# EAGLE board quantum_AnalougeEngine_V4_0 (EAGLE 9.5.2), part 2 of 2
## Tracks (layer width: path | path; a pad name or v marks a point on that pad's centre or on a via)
0,5V_DAC  (via drill 0.5)
  Top(V+) 0.508: R61.1 R60.2 52.5,40 v51.8,39.3 | IC7.3 37.84,8.06 39.1,6.79 IC7.5 41.15,6.05 41.3,5.9 v44.4,5.9
  Bottom 0.508: v51.8,39.3 51.8,13.3 v44.4,5.9
1V_DAC
  Top(V+) 0.254: IC2.7 62.35,22.5
  Top(V+) 0.305: 62.35,22.5 C23.1 | IC3.7 62.35,11.7 C24.1
  Top(V+) 0.508: C34.1 63.85,11.65 C24.1 62.3,11.75 62.3,18.7 62.5,18.9 67.3,18.9 67.3,24 67,24.3 C33.1 63.85,22.55 C23.1 | C32.1 62.35,28.15 | 62.35,28.15 62.35,22.5 | 62.35,28.15 R68.1 64.65,33.6 C20.1 R69.2 64.75,36.3 R61.2
2V_DAC_REF
  Top(V+) 0.508: R67.1 60.65,34.8 | 60.65,34.8 R68.2 | 60.65,34.8 60.62,34.77 Z1.1
+3V3_STM32  (via drill 0.5)
  Top(V+) 0.406: R1.2 100.4,56.85 100.4,85 103.8,88.4 111.9,88.4 132.3,68 163.9,68 v164,68.1
  midBottom(V-) 0.406: v164,68.1 169.7,68.1 170.2,67.6 170.2,25.6 169.5,24.9 167.12,24.9 U1.CN11_16
+5V_STM32  (via drill 0.5)
  Top(V+) 0.2: C43.1 59.3,14.65 58.6,15.35 58.6,17.6 59,18 v59.5,18
  Top(V+) 0.254: IC3.1 55.3,15 55.3,15.4 C44.1
  Top(V+) 0.305: IC2.1 55.3,25.75 55.3,26.4 C31.1
  Top(V+) 0.406: C19.1 59.4,25.75 v58,25.75 55.3,25.75 | C43.1 59.15,15 55.3,15
  pour midTop(AGND): 53.1,31.9 53.1,-1.6 173.7,-1.6 173.7,108.6 100.9,108.6 100.9,48.2 91.7,48.2 91.7,6.7 60.8,6.7 60.8,31.9
+12V  (via drill 0.5)
  Top(V+) 0.406: U$1.3 C102.1 136.95,3.85 140.25,7.15 158.35,7.15 161.4,4.1 169.9,4.1 170.4,4.6 170.4,34.3 | 165.29,35 161.5,35 160.73,34.23 U1.CN8_15 | 170.4,34.3 169.7,35 165.29,35 | 170.4,34.3 170.4,96.7 170.2,96.9 163.3,96.9 155.34,88.94 U12.9
  Top(V+) 0.508: L2.2 10.8,72.42 K2.1 12.18,73.38 v12.2,73.4 | L4.2 36.1,72.42 K3.1 35.17,73.4 v38,73.4 | L1.2 60.4,72.52 K1.1 61.78,73.38 v61.8,73.4 | L3.2 85.8,72.42 K4.1 87.38,73.38 v87.4,73.4 | K5.1 85.8,48.22 L5.2 v87.6,46.7 | L6.2 10.8,54.77 K6.1 12.13,55.73 v12.2,55.8 | L7.2 23.4,54.77 K7.1 24.67,55.73 v24.7,55.7 | L8.2 36.2,54.77 K8.1 35.27,55.7 v37.7,55.7 | v99.6,96.5 146.6,96.5 U12.9 | 165.29,35
  midBottom(V-) 0.508: v37.7,55.7 v24.7,55.7 24.6,55.8 v12.2,55.8 v12.2,73.4 v38,73.4 v61.8,73.4 v87.4,73.4 99.6,73.4 100.4,74.2 | v99.6,96.5 100.4,95.7 100.4,74.2 | 100.4,74.2 100.4,54.2 98.3,52.1 76,52.1 75.4,51.5 75.4,45.4 75.9,44.9 87.7,44.9 88.2,45.4 88.2,46.1 v87.6,46.7
.  (via drill 0.5)
  Top(V+) 0.508: IC7.7 43.09,9.34 R72.2 v43.1,11.1 | v42.95,40.25 42,40.25 R59.2
  midBottom(V-) 0.508: v43.1,11.1 43.1,21.27 43.05,21.33 43.05,40.25 v42.95,40.25
...  (via drill 0.5)
  Top(V+) 0.508: IC7.1 33.76,10.61 R71.2 33.8,10.65 v33.8,11.9 | v43.1,48.2 R73.2
  midBottom(V-) 0.508: v33.8,11.9 35.8,13.9 41.6,13.9 42,14.3 42,47.1 v43.1,48.2
ADC1-IN0  (via drill 0.5)
  Top(V+) 0.254: R4.2 R3.1 95.75,61.55 v96.8,62.6
  Bottom 0.254: v96.8,62.6 96.87,62.6 97.18,62.92
  Bottom 0.406: 97.18,62.92 116.02,62.92 116.1,63 169.1,63 169.9,62.2 169.9,40.5 169.56,40.16 166.88,40.16 165.81,39.08 U1.CN11_28
ADC1-IN3  (via drill 0.5)
  Top(V+) 0.254: R2.2 R1.1 v94.2,53.9
  Bottom 0.254: v94.2,53.9 94.2,58.8 97.6,62.2
  Bottom 0.406: 97.6,62.2 101.6,62.2 103.4,60.4 118.5,60.4 118.5,54.3 117,52.8 108.66,52.8 U1.CN12_37
AGND  (via drill 0.5)
  Top(V+) 0.254: R4.1 v98.7,60.2 | C22.2 v98.7,64.5
  Top(V+) 0.305: R6.1 R15.1 R16.1 R23.1 R24.1 | R24.1 R25.1 R26.1 R27.1 | R24.1 78.05,25.9 77.06,26.89 U$4.G6 | R39.1 v43.7,34.3 | R42.1 v43.7,30.1 | R45.1 v43.7,25.9 | R65.1 43.7,21.7 v43.7,21.6
  Top(V+) 0.406: OUT_LEFT.3 42.06,86.36 v42.1,86.4 | C12.2 38.6,80.55 | 40.65,75.25 v40.6,75.2 | TP04.P$1 CONN3.1 21.89,7.7 10.1,7.7 +15VOK.1 10,8.8 9.9,8.9 7.7,8.9 5.6,6.8 3.11,6.8 2.31,7.6 2.31,12.01 3,12.7 5,12.7 5.35,12.35 R14.2
  Top(V+) 0.508: OUT_RIGHT.3 17.57,82.77 v17.5,82.7 | C14.2 v14.2,81.5 | C13.2 16.15,75.35 v16.1,75.3 | 38.6,80.55 v38.6,82 | C11.2 40.65,75.25 | IN_LEFT.1 v88.9,82.1 | C1.2 98.5,83 v99.3,83.8 | C3.2 73.7,83.23 v74.14,83.66 | IN_RIGHT.1 v64,81.81 v64,81.8 | C4.2 v63.8,75.1 | C2.2 v88.6,75 | C6.2 88.12,67.62 | 88.12,67.62 88.8,66.95 C21.2 | 88.12,67.62 88.23,67.73 v88.7,67.73 U4.2 | C26.2 v75.15,65.85 75.25,65.75 C5.2 | U6.1 64,69 v63.9,68.9 C25.2 | v47.6,59.8 C60.2 | C62.2 48.7,63.6 | 48.7,63.6 v47.6,63.6 | C63.2 v47.6,68.1 | C61.2 48.8,55.2 | 48.8,55.2 v47.6,55.2 | 48.8,55.2 50.23,56.63 VCA2(RIGHT).6 VCA2(RIGHT).3 | 48.7,63.6 50.03,64.94 VCA1(LEFT).6 VCA1(LEFT).3 | IC8.3 54.53,46.37 v55.35,45.55 55.8,45.09 IC8.5 | C54.2 v47.8,45.5 | C53.2 v63.4,48.7 | STAGE(RIGHT).3 STAGE(RIGHT).6 25.59,38.73 25.25,38.4 C46.2 v23.5,37.5 | STAGE(LEFT).3 STAGE(LEFT).6 25.68,46.84 25.15,46.3 C47.2 v23.4,45.5 | C48.2 v23.5,50 | C45.2 v23.5,41.9 | IC5.3 30.54,29.27 v31.8,28 IC5.5 | C36.2 v23.8,28 | C30.2 3.25,34.7 v4.3,34.7 | C28.2 13.35,34.5 v14.1,34.5 | C8.2 v12.8,31.5 | U7.2 7.96,37.47 v7.9,37.4 | v17.1,42 C29.2 | C27.2 v7.5,42 | C7.2 v24.4,24.7 | U8.1 v19.6,35 | R35.1 62.45,8.6 62.45,9.9 C24.2 v63.6,9.95 65.55,9.95 C34.2 | C23.2 v63.7,20.85 65.55,20.85 C33.2 | C32.2 66.45,29.15 v66.45,32 C20.2 R69.1 66.4,35.75 66.4,35.9 67.4,36.9 67.4,39.35 66.75,40 R60.1 | TP16.P$1 56.02,34 56.8,33.23 Z1.2 | C40.2 v37,16.3 | C39.2 v37,22.2 | C57.2 v27,17.8 | C58.2 27,24.6 v26.9,24.7 | C35.2 38.9,31.8 v39,31.9 | R46.1 v43.1,50.3 | R58.1 v42.95,42.5 | C49.2 v38.2,12.2 | C50.2 v38.6,5.2 | R47.1 R76.1 R65.1
  pour midTop(AGND): 91.1,7.5 61.5,7.5 61.5,32.7 52.5,32.7 52.5,-1.7 -1,-1.7 -1,108.4 100,108.4 100,49 91.1,49
BOTTOM
  pour Bottom: -1.7,-2.6 -1.7,109.2 174.4,109.2 174.4,-2.6
BUSY
  Top(V+) 0.406: U$4.BUSY 97.61,18 99.9,18 102.9,21 102.9,23.9 103.9,24.9 109.3,24.9 109.8,25.4 109.8,27.3 111.2,28.7 116.1,28.7 118.05,30.65 126.69,30.65 153.94,57.9 163.06,57.9 164.31,59.15 U1.CN11_44
CHASIS  (via drill 0.5)
  Top(V+) 0.406: C15.1 67.8,85.15 v67.8,88 | C18.1 92.75,87.85 v92.6,88
  Top(V+) 1.016: R77.1 50.3,7.9 48.9,6.5 TP03.P$1
  Bottom 1.016: 82.69,88 v92.6,88 | 82.69,88 73.89,96.8 40.2,96.8 OUT2(L/M).G OUT1(R/S).G 5.4,94.8 1.5,90.9 1.5,55.6 6.11,50.99 6.11,45.81 1.9,41.6 1.9,12.6 11.6,2.9 46.8,2.9 TP03.P$1 | 82.69,88 v67.8,88
CS  (via drill 0.5)
  Top(V+) 0.406: U$4.CS 100.53,16.73 103.6,19.8 109.3,19.8 110.6,21.1 110.6,25.3 111.4,26.1 115.7,26.1 119.34,29.74 127.14,29.74 152.7,55.3 162.2,55.3 163.1,56.2 v163.1,57
  Bottom 0.406: v163.1,57 163.1,59 164.46,60.36 167.08,60.36 168.35,61.64 U1.CN11_45
CS_DAC1  (via drill 0.5)
  Top(V+) 0.254: IC2.9 57.9,23.5 v57.3,24.1
  midBottom(V-) 0.305: v57.3,24.1 58,23.4 58,21.3 56.7,20 56.7,6.39 58.39,4.7
  midBottom(V-) 0.406: 58.39,4.7 93.01,4.7 93.88,5.57 93.88,11.98 94.9,13 99.5,13 102.7,16.2 102.7,31.8 103.4,32.5 109.9,32.5 110.8,33.4 110.8,41.4 109.6,42.6 103.4,42.6 102.9,42.1 102.9,40.5 103.3,40.1 106.4,40.1 107.39,39.11 U1.CN12_27
CS_DAC2  (via drill 0.5)
  Top(V+) 0.254: IC3.9 57.8,12.7 v57.4,13.1
  midBottom(V-) 0.305: v57.4,13.1 57.4,7 59,5.4
  midBottom(V-) 0.406: U1.CN12_29 109.13,41.37 109.6,40.9 109.6,35.9 108.8,35.1 103.8,35.1 101.6,32.9 101.6,17.6 99.5,15.5 93.9,15.5 92.9,14.5 92.9,5.9 92.4,5.4 59,5.4
CV_A_B
  Bottom 0.406: U1.CN11_3 168.35,8.55 167.3,9.6 163.7,9.6 159.91,13.39 111.01,13.39 109.7,14.7 101.54,14.7 99.81,12.96 97.65,12.96 U$4.CVB U$4.CVA
DAC2_OUT1(OFFSET_VCA1)  (via drill 0.5)
  Top(V+) 0.508: R76.2 R74.2 48.2,19.75 v48.2,21 | C39.1 v40.4,22.3 | v26.9,20.1 26.43,20.57 IC9.3
  Bottom 0.508: v48.2,21 46.95,22.25 40.45,22.25 v40.4,22.3 38.2,20.1 v26.9,20.1
DAC2_OUT2(OFFSET_VCA2)  (via drill 0.5)
  Top(V+) 0.508: R47.2 R75.2 48.1,17.45 v48.1,15.8 | v40.4,16.5 C40.1 38.8,19.9 35.6,19.9 34.99,19.3 IC9.5
  Bottom 0.508: v40.4,16.5 40.5,16.6 47.3,16.6 v48.1,15.8
DAC2_OUT3
  Top(V+) 0.254: IC3.4 45.8,11.7 43.9,13.6 34.65,13.6 R62.1
DAC2_OUT4
  Top(V+) 0.254: IC3.5 45.75,11.2 45.3,10.75 R70.1
DAC_OUT1  (via drill 0.5)
  Top(V+) 0.508: R57.1 18.25,23.05 v18.2,23
  midBottom(V-) 0.406: v18.2,23 18.2,20.2 27.5,10.9 27.5,3.8 29.6,1.7 116.1,1.7 157.1,42.7 164.6,42.7 U1.CN11_32
DAC_OUT2  (via drill 0.5)
  Top(V+) 0.508: R55.1 34.85,22.25 v34.9,22.3
  midTop(AGND) 0.406: v110.3,5.8 110.3,17.6 109.39,18.51 U1.CN12_11
  midBottom(V-) 0.406: v34.9,22.3 34.9,16.7 29.1,10.9 29.1,3.9 30.1,2.9 107.5,2.9 110.3,5.7 v110.3,5.8
DB0
  midBottom(V-) 0.406: U$4.DB0 97.57,20.5 94.8,20.5 94.2,21.1 94.2,42.94 97.51,46.25 102.05,46.25 102.7,46.9 102.7,83.5 103.75,84.55 U1.CN12_64 105.41,84.55 106.69,83.27 109.63,83.27 115.01,77.89 U1.CN10_33
DB1
  midBottom(V-) 0.406: U$4.DB1 97.6,23.07 97.6,43.1 99.7,45.2 126.6,45.2 164.7,83.3 167.06,83.3 U1.CN11_61
DB2
  midTop(AGND) 0.406: U$4.DB2 101.25,24.35 102.2,25.3 102.2,26.9 102.69,27.39 108.89,27.39 109.67,28.16 109.67,31.77 110.2,32.3 117,32.3 117,63.7 116.47,64.23 U1.CN10_25 145.53,64.23 155.69,54.07 U1.CN9_14
DB3
  Top(V+) 0.406: U$4.DB3 97.59,25.6 99.9,25.6 100.7,26.4 100.7,28.7 101.9,29.9 108.6,29.9 109.1,30.4 109.1,31.6 109.8,32.3 124.3,32.3 156.3,64.3 158.12,64.3 U1.CN9_22 159.46,65.5 167.08,65.5 U1.CN11_47
DB4
  Bottom 0.406: U$4.DB4 102.01,26.89 104,24.9 109.1,24.9 110.6,26.4 110.6,28.1 111.24,28.74 116.14,28.74 117.94,30.54 126.54,30.54 152.6,56.6 U1.CN9_16
DB5
  Bottom 0.406: U$4.DB5 96.34,26.9 97.56,28.12 102.5,28.12 103.18,27.44 109.04,27.44 109.8,28.2 109.8,30.5 110.75,31.45 126.09,31.45 153.79,59.15 U1.CN9_18
DB6
  midBottom(V-) 0.406: U1.CN9_20 159.5,63 162.8,63 162.8,79.8 165.01,82.01 U1.CN11_62
  Bottom 0.406: U$4.DB6 98.93,29.43 99.4,29.9 108.5,29.9 109,30.4 109,31.8 109.6,32.4 125.8,32.4 155.1,61.7 U1.CN9_20
DB7
  Bottom 0.406: U$4.DB7 97.51,30.6 100.2,30.6 101.3,31.7 101.3,59.4 104.6,59.4 U1.CN12_44 106.1,57.9 111.18,57.9 U1.CN10_20
DB8
  midTop(AGND) 0.406: U$4.DB8 102.9,35.99 102.9,55.3 111.24,55.3 U1.CN10_18
DB9  (via drill 0.5)
  Top(V+) 0.406: U$4.DB9 97.57,33.2 100.4,33.2 101,33.8 101,36.4 102.2,37.6 111.16,37.6 U1.CN10_4 112.47,36.47 113.6,37.6 117.6,37.6 118.7,38.7 v118.7,47.1
  midBottom(V-) 0.406: U1.CN12_52 105.29,69.31 106.6,68 115.8,68 118.6,65.2 118.6,47.2 v118.7,47.1
DB10
  midTop(AGND) 0.406: U$4.DB10 102,37.63 102,65.51 106.11,65.51 U1.CN12_47 109.83,64.23 112.37,61.69 U1.CN10_24
DB11
  Top(V+) 0.406: U1.CN10_6 112.47,38.84 111.16,40.16 101.56,40.16 101.1,39.7 101.1,37.4 99.44,35.74 97.57,35.74 U$4.DB11
DB12
  midTop(AGND) 0.406: U$4.DB12 101.3,39.47 101.3,68.1 106.06,68.1 107.28,66.88 | 107.28,66.88 U1.CN12_49 | U1.CN10_26 109.82,66.88 107.28,66.88
DB13
  Top(V+) 0.406: U$4.DB13 97.55,38.26 99.31,38.26 100.3,39.26 100.3,44.7 100.84,45.24 111.14,45.24 U1.CN10_10 112.47,44.06 113.64,45.24 116.94,45.24 117.8,46.1 117.8,74.3 115.7,76.4 109.4,76.4 U1.CN12_55
DB14
  Top(V+) 0.406: U$4.DB14 98.88,44.79 102.05,47.96 102.05,69.9 102.69,70.54 106.16,70.54 U1.CN12_51 107.45,69.37 109.87,69.37 U1.CN10_28
DB15
  Top(V+) 0.406: U$4.DB15 96.34,43.39 101.4,48.45 101.4,71.6 102.98,73.18 106.06,73.18 U1.CN12_53
DGND
  pour Top(V+): 53.1,31.9 53.1,-1.2 173.4,-1.2 173.4,108.6 100.9,108.6 100.9,48.2 91.7,48.2 91.7,6.6 61.1,6.6 61.1,31.9
  pour midBottom(V-): 53,31.9 53,-2.1 174.1,-2.1 174.1,108.6 100.9,108.6 100.9,48.2 91.7,48.2 91.7,6.6 60.8,6.6 60.8,31.9
DIN_DAC  (via drill 0.5)
  Top(V+) 0.254: IC3.8 58.4,12.2 56.1,9.9 v56.1,9.8
  Top(V+) 0.305: IC2.8 57.8,23 v57.2,22.4
  midBottom(V-) 0.305: v57.2,22.4 56.1,21.3 v56.1,9.8 56.1,5.7 57.8,4
  midBottom(V-) 0.406: 57.8,4 93.6,4 94.8,5.2 94.8,10.1 95,10.3 99.5,10.3 103.9,14.7 109.8,14.7 110.8,15.7 110.8,17.8 111.5,18.5 129.7,18.5 156.4,45.2 160.1,45.2 160.73,44.57 U1.CN9_5
E+_OUT_STAGE_LEFT
  Top(V+) 0.508: STAGE(LEFT).2 37.77,45.56 38.3,46.1 TP02.P$1 40.05,48.8 40.15,48.9 | R46.2 40.15,48.9 | 40.15,48.9 R73.1
E+_OUT_STAGE_RIGHT
  Top(V+) 0.508: STAGE(RIGHT).2 37.27,37.47 38.2,38.4 TP01.P$1 39.95,41 40.15,41.2 | R58.2 40.15,41.2 | 40.15,41.2 R59.1
EC+_VCA1(LFT)  (via drill 0.5)
  Top(V+) 0.508: VCA1(LEFT).2 60.06,63.66 60.85,64.45 TP37.P$1 60.85,68.55 60,69.4 v45,69.4 | R56.2 24.09,23.05 IC9.1 26.2,23.11 v27.4,21.9
  Bottom 0.508: v27.4,21.9 30.5,21.9 33.19,24.59 33.19,48.19 43.7,58.7 43.7,68.1 v45,69.4
EC+_VCA2(RIGHT)  (via drill 0.5)
  Top(V+) 0.508: VCA2(RIGHT).2 59.97,55.37 60.85,56.25 TP36.P$1 57.95,60.8 v45.5,60.8 | IC9.7 31.39,21.84 R54.2 33.15,23.6 v34.2,23.6
  Bottom 0.508: v34.2,23.6 34.2,47.7 44.7,58.2 44.7,60.4 45.1,60.8 v45.5,60.8
FRST
  Top(V+) 0.406: U$4.FRST 97.67,20.6 100.4,20.6 101.6,21.8 101.6,26 103,27.4 108.5,27.4 109.9,28.8 109.9,30.7 110.7,31.5 126,31.5 154.88,60.38 167.62,60.38 168.35,59.65 U1.CN11_43
L  (via drill 0.5)
  Top(V+) 0.508: IN_LEFT.6 IN_LEFT.5 96.2,72.9 95.3,72 90.92,72 88.77,69.85 82.92,69.85 82.4,69.33 v82.4,68.3 82.45,68.3 82.45,67.33 82.64,67.14 IC4.3 | v82.4,54.3 84.9,54.3 K5.Q1
  Bottom 0.508: v82.4,68.3 v82.4,54.3
L/M_IN(VCA1_IN)
  Top(V+) 0.508: C67.1 71.8,60.7 74.4,58.1 80.7,58.1 82,56.8 K5.P1 88,56.8 90.2,54.6 90.2,42.55 87.25,39.6 R5.1
L/M_OUT(OUT_STAGE_LEFT)  (via drill 0.5)
  Top(V+) 0.305: R19.1 88.3,25.9 90.3,23.9 90.3,13.7 88.1,11.5 71.5,11.5 68.3,14.7 68.3,40.4 67.4,41.3 47.4,41.3 40.1,34 28.7,34 26.8,32.1 R28.2
  Top(V+) 0.508: IC5.1 27.36,31.8 R28.2 C37.2 23.95,31.25 | IC1.3 18.86,29.54 19.3,29.1 21.8,29.1 23.95,31.25 | 23.95,31.25 22.4,32.8 v22.4,35.3 | v9.8,59.2 9.8,60.86 K6.Q1
  Bottom 0.508: v22.4,35.3 15.4,42.3 15.4,59.2 v9.8,59.2
L/M_OUT(VCA1_OUT)  (via drill 0.5)
  Top(V+) 0.508: 52.5,48.91 50.76,48.91 R48.2 C55.2 48.6,48.85 45.55,48.85 43.9,47.2 43.9,45.5 42.7,44.3 R36.1 | 52.5,48.91 IC8.1 | R17.1 86.55,32.8 88.5,34.75 v88.5,37.9 | v52.6,50.1 52.6,49.01 52.5,48.91
  Bottom 0.508: v88.5,37.9 88.5,41.2 86.6,43.1 54.1,43.1 52.6,44.6 v52.6,50.1
L/M_OUT+
  Top(V+) 0.508: K3.S1 36.66,83.64 37.4,82.9 37.4,75.6 39,74 44.6,74 OUT_LEFT.8 | OUT_LEFT.8 OUT_LEFT.7 | OUT_LEFT.8
L/M_OUT-
  Top(V+) 0.508: K3.S2 30.14,83.64 33.9,87.4 44,87.4 44,84.6 | OUT_LEFT.2 44,84.6 | 44,84.6 OUT_LEFT.1
M
  Top(V+) 0.508: U4.5 U4.6 96.3,63.52 92.12,59.34 K5.S1
M1  (via drill 0.5)
  Top(V+) 0.508: U7.6 U7.5 v4.6,42.4 | K6.S1 7.99,65.99 v7.6,65.6
  Bottom 0.508: v7.6,65.6 8.8,64.4 8.8,44.5 6.7,42.4 v4.6,42.4
N$1
  Top(V+) 0.406: C9.1 63.05,81.25 63.77,80.53 IN_RIGHT.2
  Top(V+) 0.508: C9.1 63.05,83.64 K1.S1
N$2
  Top(V+) 0.508: K1.S2 53.36,83.64 57.2,79.8 63,79.8 63.53,79.27 IN_RIGHT.3 68.3,79.27 68.3,81.3 69.9,82.9 72.03,82.9 73.45,84.33 73.45,84.6 C10.2
N$3
  Top(V+) 0.406: C9.2 66.35,83.5 69.2,83.5 69.55,83.85 C15.2 C10.1
N$4  (via drill 0.5)
  Top(V+) 0.305: U$4.V1 72.24,39.59 73.59,40.94 75.51,40.94 76.5,39.95 76.5,38.65 v76.35,38.5 | v83.1,38 83.1,38.95 | 83.1,38.95 R5.2 | 83.1,38.95 82.45,39.6 R6.2
  Bottom 0.305: v76.35,38.5 82.6,38.5 v83.1,38
N$5
  Top(V+) 0.508: K8.Q1 33.13,60.91 30.23,58 29.1,58 26,58 24.4,59.6 19.97,59.6 18.99,60.58 18.99,66 | 18.99,66 22.43,66 K7.S1 | 18.99,66 18.99,66.01 17.55,67.45 8.05,67.45 6.6,66 6.6,64.1 7.25,63.45 K6.P1
N$6  (via drill 0.5)
  Top(V+) 0.305: U$4.V2 71.34,37.05 70.96,37.43 70.96,40.25 72.36,41.65 75.9,41.65 77.2,40.34 77.2,34.95 v77.06,34.8 | v83.1,34.4 83.1,35.75 | 83.1,35.75 83.05,35.7 R15.2 | 83.1,35.75 R13.2
  Bottom 0.305: v77.06,34.8 82.7,34.8 v83.1,34.4
N$7
  Top(V+) 0.508: K4.S2 79.78,83.64 80.4,83.02 80.4,80.7 81.21,79.89 88.51,79.89 88.9,79.5 90.94,79.5 IN_LEFT.3 93.06,79.56 93.9,80.4 93.9,82.5 95,83.6 97.33,83.6 98.65,84.92 C17.2
N$8  (via drill 0.5)
  Top(V+) 0.508: K2.Q1 7.66,78.56 v6.7,77.6 | v59.25,76.45 59.25,78.26 K1.Q1
  Bottom 0.508: v6.7,77.6 14.9,77.6 58.2,77.6 59.3,76.5 v59.25,76.45
N$9
  Top(V+) 0.406: C17.1 C18.2 94.45,84.3 94.25,84.1 91.95,84.1 90.95,85.1 C16.2
N$10  (via drill 0.5)
  Top(V+) 0.305: U$4.V3 70.84,34.51 70.35,34.99 70.35,40.64 72.06,42.35 76.39,42.35 77.91,40.84 77.91,31.45 v77.76,31.3 | v83.1,30.9 83.1,32.05 | 83.1,32.05 83.1,32.15 R17.2 | 83.1,32.05 R16.2
  Bottom 0.305: v77.76,31.3 82.7,31.3 v83.1,30.9
N$11  (via drill 0.5)
  Top(V+) 0.508: K2.Q2 4.51,76.6 v9.8,76.6 | v52,76.6 52,78.3 K1.Q2
  Bottom 0.508: v9.8,76.6 v52,76.6
N$12  (via drill 0.5)
  Top(V+) 0.305: U$4.V4 70.98,31.97 69.65,33.3 69.65,40.93 71.77,43.06 76.99,43.06 78.61,41.43 78.61,28.21 v78.3,27.9 | v83.1,27.5 83.1,28.75 | 83.1,28.75 R18.2 | 83.1,28.75 82.45,29.4 R23.2
  Bottom 0.305: v78.3,27.9 82.7,27.9 v83.1,27.5
N$13
  Top(V+) 0.406: C16.1 88.05,85.1 87.95,85 87.95,81.35 88.5,80.8 90.97,80.8 IN_LEFT.2
  Top(V+) 0.508: C16.1 85.2,85.1 84.84,84.75 K4.S1
N$14
  Top(V+) 0.508: L1.1 53.25,71.3 R7.2
N$15  (via drill 0.5)
  Top(V+) 0.508: v32,81.1 K3.P1
  Bottom 0.508: OUT2(L/M).3 32,83.52 v32,81.1
N$16
  Top(V+) 0.508: R8.2 84.1,71.1 L3.1
N$17  (via drill 0.5)
  Top(V+) 0.508: K3.P2 v30.4,81.1
  Bottom 0.508: v30.4,81.1 30.4,85.73 OUT2(L/M).2
N$18  (via drill 0.5)
  Top(V+) 0.508: U4.3 92.64,66.47 93.4,65.7 93.4,64.5 92.1,63.2 84.75,63.2 84.05,63.9 IC4.1 IC4.2 81.83,65.86 81.05,66.65 81.05,68.8 80.45,69.4 v76.6,69.4 | U6.2 66.23,67.7 v67.9,67.7
  Bottom 0.508: v76.6,69.4 69.6,69.4 v67.9,67.7
N$19
  Top(V+) 0.508: K8.S1 32.84,65.99 32.24,65.39 32.24,61.39 29.96,59.11 26.25,59.11 24.45,60.91 K7.Q1 20.39,60.91 20,61.3 20,64.1 20.66,64.75 24.29,64.75 24.69,65.15 24.69,67 24.4,67.29 19.05,67.29 17.93,68.4 7.72,68.4 5.6,66.28 5.6,64.2 4.85,63.45 K6.P2
N$20  (via drill 0.5)
  Top(V+) 0.305: U$4.V5 70.94,29.43 69.65,28.14 69.65,15.87 71.77,13.74 76.59,13.74 78.3,15.46 v78.3,24.4 | v83.1,24 83.1,25.25 | 83.1,25.25 R19.2 | 83.1,25.25 82.45,25.9 R24.2
  Bottom 0.305: v83.1,24 82.7,24.4 v78.3,24.4
N$21
  Top(V+) 0.508: IN1(R/S).2 65.64,92.5 57.12,92.5 55.49,90.88 55.49,86.49 54.1,85.1 50.71,85.1 49.8,84.19 49.8,81.6 50.3,81.1 K1.P2
N$22
  Top(V+) 0.508: IN1(R/S).3 57.95,90.35 57.1,89.5 57.1,81.6 57.6,81.1 K1.P1
N$23  (via drill 0.5)
  Top(V+) 0.508: v5.6,81.1 K2.P2
  Bottom 0.508: OUT1(R/S).2 5.6,86.13 v5.6,81.1
N$24  (via drill 0.5)
  Top(V+) 0.508: v6.9,81.1 K2.P1
  Bottom 0.508: OUT1(R/S).3 6.9,83.62 v6.9,81.1
N$25
  Top(V+) 0.508: IN2(L/M).3 83.55,90.35 82.5,89.3 82.5,81.5 82.9,81.1 K4.P1
N$26
  Top(V+) 0.508: R12.2 L8.1
N$27
  Top(V+) 0.508: IN2(L/M).2 91.14,92.7 83.2,92.7 81.4,90.9 81.4,86.4 80.2,85.2 76.1,85.2 75.2,84.3 75.2,81.8 75.9,81.1 K4.P2
N$28  (via drill 0.5)
  Top(V+) 0.508: K3.Q1 35.15,79.39 v35.4,79.65 | v84.8,76.1 84.8,78.51 K4.Q1
  Bottom 0.508: v35.4,79.65 39.25,79.65 39.3,79.7 73.3,79.7 76.9,76.1 v84.8,76.1
N$29
  Top(V+) 0.508: R11.2 L7.1
N$30
  Top(V+) 0.508: R10.2 L6.1
N$31  (via drill 0.5)
  Top(V+) 0.508: K3.Q2 31.45,78.56 v31.5,78.6 | K4.Q2 77.5,78.5 v77.5,77.1
  Bottom 0.508: v31.5,78.6 33.6,80.7 73.9,80.7 v77.5,77.1
N$32
  Top(V+) 0.508: R9.2 L5.1
N$33  (via drill 0.5)
  Top(V+) 0.508: IC4.7 IC4.6 | U4.1 93.19,69 94.31,67.89 94.31,63.91 92.69,62.29 84.11,62.29 80.53,65.86 IC4.7 | IC4.7 78.55,67.17 76.64,67.17 v76.6,67.2 | v68.1,66.4 66.27,66.4 U6.3
  Bottom 0.508: v76.6,67.2 68.9,67.2 v68.1,66.4
N$34  (via drill 0.5)
  Top(V+) 0.305: U$4.V6 70.94,26.89 70.25,26.2 70.25,16.56 72.36,14.45 75.89,14.45 77.51,16.07 77.51,20.99 v77.5,21 | v83.1,20.6 83.1,21.85 | 83.1,21.85 R20.2 | 83.1,21.85 82.45,22.5 R25.2
  Bottom 0.305: v77.5,21 82.8,21 83.1,20.7 v83.1,20.6
N$35  (via drill 0.5)
  Top(V+) 0.305: U$4.V7 71.34,24.35 70.86,23.87 70.86,17.25 72.86,15.25 75.4,15.25 76.81,16.66 76.81,17.55 v76.76,17.6 | v83.1,17.2 83.1,18.45 | 83.1,18.45 R21.2 | 83.1,18.45 82.45,19.1 R26.2
  Bottom 0.305: v76.76,17.6 82.7,17.6 v83.1,17.2
N$36  (via drill 0.5)
  Top(V+) 0.305: v75.2,16.35 v75.19,16.36 72.89,16.36 71.61,17.64 71.61,21.21 U$4.V8 | v83.1,13.7 83.1,14.85 | 83.1,14.85 R22.2 | 83.1,14.85 82.45,15.5 R27.2
  Bottom 0.305: v75.2,16.35 75.2,14.75 75.95,14 82.9,14 83.1,13.8 v83.1,13.7
N$43
  Top(V+) 0.508: IC1.7 IC1.6 18.85,26.53 18.85,25.53 18.47,25.15 17.02,25.15 16.64,25.53 16.64,29.46 16.1,30 11.6,30 11.6,32.99 | U7.1 9.8,34.8 11.6,32.99 | U8.3 17.7,38.73 17.7,35 16,33.3 11.6,33.3 11.6,32.99
N$45  (via drill 0.5)
  Top(V+) 0.508: IC1.2 IC1.1 v21.41,34.3 21.41,37.12 21.07,37.45 19.62,37.45 U8.2 | v7.8,38.8 9.73,38.8 U7.3
  Bottom 0.508: v21.41,34.3 20.41,33.3 10.1,33.3 10.1,38.1 9.4,38.8 v7.8,38.8
N$48  (via drill 0.5)
  Top(V+) 0.508: STAGE(LEFT).8 30.61,44.3 v30.9,44 | v30.7,30.5 28.89,30.5 IC5.2 28.06,30.54 27.07,29.55 R28.1 25.5,29.55 C37.1
  Bottom 0.508: v30.9,44 30.9,30.7 v30.7,30.5
N$49
  Top(V+) 0.508: L2.1 R33.2
N$50
  Top(V+) 0.406: R14.1 3.65,8.05
  Top(V+) 0.508: 3.65,8.05 -15VOK.2
N$51
  Top(V+) 0.508: L4.1 R34.2
N$52
  Top(V+) 0.406: R29.1 8.35,12.35 7,13.7 2.3,13.7 1.3,12.7 1.3,7.4 2.7,6 7.4,6 8.4,7 +15VOK.2
N$53  (via drill 0.5)
  Top(V+) 0.508: STAGE(RIGHT).8 v32,36.2 | v32.3,29.3 34.31,29.3 | 34.31,29.3 IC5.6 | C38.1 R30.1 36.02,28.55 35.27,29.3 34.31,29.3
  Bottom 0.508: v32,36.2 32,29.6 v32.3,29.3
N$54
  Top(V+) 0.508: C45.1 R32.2 STAGE(RIGHT).5
N$55
  Top(V+) 0.508: R36.2 STAGE(LEFT).1
N$56
  Top(V+) 0.254: R38.2 51.5,34.75 51.5,25.68 51.91,25.28 51.91,24.03 52.47,23.47 55.3,23.47 IC2.2
N$57
  Top(V+) 0.254: R41.2 50.35,32.2 50.8,31.75 50.8,25.34 51.25,24.89 51.25,23.55 51.78,23.02 55.28,23.02 IC2.3
N$58
  Top(V+) 0.254: R44.2 49.85,25.25 50.6,24.5 50.7,24.4 50.7,23 51.2,22.5 IC2.4
N$59
  Top(V+) 0.254: IC2.5 50.9,22 49.85,23.05 R64.2
N$60
  Top(V+) 0.254: IC3.2 51.6,12.7 50.8,13.5 50.8,19.6 R74.1
N$61
  Top(V+) 0.254: IC3.3 51.2,12.2 49.85,13.55 49.85,17.5 R75.1
N$63
  Top(V+) 0.508: R57.2 R56.1 22.29,21.84 IC9.2
N$64  (via drill 0.5)
  Top(V+) 0.508: C55.1 R48.1 51.15,47.05 51.73,47.63 IC8.2 54.23,47.63 v54.3,47.7 | VCA1(LEFT).8 v54.49,62.4 v54.5,62.4
  Bottom 0.508: v54.5,62.4 54.9,62 54.9,48.3 v54.3,47.7
N$65
  Top(V+) 0.508: R52.2 61.7,60.7 60,62.4 VCA1(LEFT).1
N$68
  Top(V+) 0.508: STAGE(RIGHT).1 R37.2
N$71
  Top(V+) 0.508: C67.2 R52.1
N$72
  Top(V+) 0.508: R62.2 R71.1 34.19,9.34 IC7.2
N$73
  Top(V+) 0.508: C48.1 R31.2 STAGE(LEFT).5
N$74
  Top(V+) 0.508: IC7.6 42.69,8.06 R72.1 R70.2
N$75  (via drill 0.5)
  Top(V+) 0.508: C56.1 R49.1 60.12,45.45 59.23,46.34 58.27,46.34 IC8.6 58.22,46.4 v56.4,46.4 | VCA2(RIGHT).8 v55.85,54.09 v55.85,54.1
  Bottom 0.508: v55.85,54.1 56.15,53.8 56.15,46.65 v56.4,46.4
N$77
  Top(V+) 0.508: VCA2(RIGHT).5 R51.2 C60.1
N$78
  Top(V+) 0.508: C68.2 R53.1
N$79
  Top(V+) 0.508: R53.2 61.4,55.1 60.4,54.09 VCA2(RIGHT).1
N$80
  Top(V+) 0.508: VCA1(LEFT).5 R50.2 C63.1
N$81
  Top(V+) 0.508: IC9.6 31.79,20.57 R54.1 R55.2
OS0
  Bottom 0.406: U$4.OS0 100.49,6.57 101.25,5.81 U1.CN12_2
OS1
  Bottom 0.406: U$4.OS1 97.57,7.8 100.4,7.8 101.06,7.14 106.12,7.14 107.39,5.86 U1.CN12_1
OS2
  Bottom 0.406: U$4.OS2 99.37,9.6 110.2,9.6 111.39,8.41 116.4,8.41 117.51,7.3 162.5,7.3 163.4,6.4 163.4,5.2 164.6,4 167.9,4 168.35,4.45 U1.CN11_1
OUT1_DRIVER  (via drill 0.5)
  Top(V+) 0.508: R33.1 1.75,72.57 K2.2 2.6,73.42 v2.6,74.9 | K1.2 51.35,72.47 R7.1 47.7,71.1 v47.7,103.6 | v148.3,80.1 154.12,80.1 U12.16
  midBottom(V-) 0.508: v2.6,74.9 2.6,102.2 49.1,102.2 | 49.1,102.2 v47.7,103.6 | v148.3,80.1 146.3,82.1 146.3,98.1 142.2,102.2 49.1,102.2
OUT2_DRIVER  (via drill 0.5)
  Top(V+) 0.508: K3.2 26.95,72.47 R34.1 26.9,71.05 v26.9,69.8 | K4.2 76.75,72.57 R8.1 v75.3,71.1 | v145.72,81.33 U12.15 | U12.15 | v46.7,95.4 v46.7,71.1
  midBottom(V-) 0.508: v26.9,69.8 28.2,71.1 v46.7,71.1 v75.3,71.1 | v46.7,95.4 46.7,95.9 47.6,96.8 93,96.8 95.4,99.2 141.1,99.2 143.44,96.86 143.44,83.68 145.72,81.39 v145.72,81.33
OUT3_DRIVER  (via drill 0.5)
  Top(V+) 0.508: R9.1 76.75,48.17 K5.2 77.66,50.35 v78.2,50.9 | v143.18,82.58 154.15,82.58 U12.14
  midBottom(V-) 0.508: v78.2,50.9 98.6,50.9 101.5,53.8 101.5,96.3 103.3,98.1 140.9,98.1 142.53,96.47 142.53,83.3 143.18,82.65 v143.18,82.58
OUT4_DRIVER  (via drill 0.5)
  Top(V+) 0.508: R10.1 1.75,54.92 K6.2 2.6,55.77 v2.6,57.1 | v145.35,83.9 154.12,83.9 U12.13
  midBottom(V-) 0.508: v2.6,57.1 2.6,72.2 3.6,73.2 3.6,101.19 141.9,101.19 145.35,97.75 v145.35,83.9
OUT5_DRIVER  (via drill 0.5)
  Top(V+) 0.508: K7.2 14.25,54.82 R11.1 12.65,53.35 v12.6,53.3 | v144.39,85.1 154.12,85.1 U12.12
  midBottom(V-) 0.508: v12.6,53.3 4.5,53.3 3.6,54.2 3.6,71.7 4.6,72.7 4.6,100.2 141.6,100.2 144.39,97.41 v144.39,85.1
OUT6_DRIVER  (via drill 0.5)
  Top(V+) 0.508: K8.2 27.05,54.82 R12.1 25.55,53.35 v23.9,51.7 | v147.3,86.4 U12.11
  midBottom(V-) 0.508: v23.9,51.7 4.4,51.7 1.4,54.7 1.4,105.4 86,105.4 88.1,103.3 142.48,103.3 147.3,98.48 v147.3,86.4
OUT_L/M
  Top(V+) 0.508: OUT_LEFT.4 40.8,83.31 41.6,82.5 43.9,82.5 45.6,80.8 45.6,73.6 44.9,72.9 40.3,72.9 37.4,70 37.4,64.1 36.75,63.45 K8.P1
OUT_R/S
  Top(V+) 0.508: OUT_RIGHT.4 16.3,82.5 17.5,81.3 22.1,81.3 25.6,77.8 25.6,63.85 25.2,63.45 K7.P1
R  (via drill 0.5)
  Top(V+) 0.508: IN_RIGHT.6 71.4,78.3 IN_RIGHT.5 73.41,78 74.35,77.05 74.35,70.25 76.19,68.41 IC4.5 v80.1,68.4 | K5.Q2 80.06,54.26 v80.1,54.3
  Bottom 0.508: v80.1,68.4 v80.1,54.3
R/S_IN(VCA2_IN)  (via drill 0.5)
  Top(V+) 0.508: K5.P2 74.5,56.8 | 74.5,56.8 72.8,55.1 C68.1 | R13.1 86.15,36.4 87,37.25 v87,37.9 | v86.95,40.95 89.19,43.19 89.19,50.9 87.39,52.7 74.5,52.7 74.5,56.8
  Bottom 0.508: v87,37.9 87,40.9 v86.95,40.95
R/S_OUT(OUT_STAGE_RIGHT)  (via drill 0.5)
  Top(V+) 0.305: R20.1 87.9,22.5 89.35,21.05 89.35,14.35 87.7,12.7 71.5,12.7 69,15.2 69,40.7 67.7,42 47.1,42 39.9,34.8 v39.8,34.8
  Top(V+) 0.508: IC5.7 35.41,30.54 35.7,30.25 R30.2 C38.2 38.7,29.75 38.97,29.75 v39.35,29.37 39.35,27.73 37.52,25.9 v24.2,25.9 24.1,25.9 21.9,28.1 17.6,28.1 17.59,28.09 IC1.5 | K6.Q2 2.56,59.45 3.9,58.1 v18.6,58.1
  Bottom 0.305: v39.35,29.37 39.8,29.82 v39.8,34.8
  Bottom 0.508: v24.2,25.9 25,26.7 25,34.45 20.1,39.35 20.1,56.6 v18.6,58.1
R/S_OUT(VCA2_OUT)  (via drill 0.5)
  Top(V+) 0.508: IC8.7 59.16,47.63 59.65,47.15 R49.2 C56.2 63.17,47.15 63.7,46.62 63.7,44.4 v63.44,44.14 63.44,44.01 62.18,42.75 46.8,42.75 40.25,36.2 R37.1 | R18.1 87.55,29.4 90,31.85 v90,37.9
  Bottom 0.508: v90,37.9 90,41.7 87.56,44.14 v63.44,44.14
R/S_OUT+
  Top(V+) 0.508: K2.S1 9.98,83.5 11.92,83.5 12.4,83.02 12.4,76.1 14.5,74 20.1,74 OUT_RIGHT.8 | OUT_RIGHT.8 | OUT_RIGHT.7 OUT_RIGHT.8
R/S_OUT-
  Top(V+) 0.508: K2.S2 4.64,83.64 7.3,86.3 19.4,86.3 19.5,86.2 19.5,84.4 | 19.5,84.4 OUT_RIGHT.1 | 19.5,84.4 OUT_RIGHT.2
RANGE
  Bottom 0.406: U$4.RANGE 97.63,10.4 101.1,10.4 102.8,12.1 109.7,12.1 110.9,10.9 160.72,10.9 U1.CN11_2
RD
  Top(V+) 0.406: U$4.RD 97.67,15.52 101.91,15.52 102.72,14.7 110.2,14.7 111.5,13.4 159.26,13.4 164.31,8.35 U1.CN11_4
RELAIS1
  Top(V+) 0.406: U12.1 162.04,80.06 165.16,76.93 U1.CN11_58
RELAIS2
  Top(V+) 0.406: U12.2 162.3,81.33 162.94,80.68 167.14,80.68 U1.CN11_59
RELAIS3
  Top(V+) 0.406: U12.3 163.85,82.59 U1.CN11_64
RELAIS4  (via drill 0.5)
  Top(V+) 0.406: U12.4 160.68,83.9 v163.6,83.9
  Bottom 0.406: v163.6,83.9 163.6,87 163.9,87.3 165.6,87.3 U1.CN11_66
RELAIS5  (via drill 0.5)
  Top(V+) 0.406: U12.5 162.44,85.14 v162.5,85.2
  Bottom 0.406: v162.5,85.2 162.5,87.1 163.8,88.4 167.7,88.4 168.35,87.75 U1.CN11_65
RELAIS6
  Top(V+) 0.406: U12.6 162.4,86.41 162.94,85.86 167.04,85.86 U1.CN11_63
RESET
  Bottom 0.406: U$4.RST 102,17.31 102,21 103.3,22.3 110,22.3 111.3,23.6 123.5,23.6 155.2,55.3 164.5,55.3 U1.CN11_42
S
  Top(V+) 0.508: U6.6 U6.5 77.26,59.34 K5.S2
S1  (via drill 0.5)
  Top(V+) 0.508: U8.6 U8.5 14.4,45.1 v7.5,45.1 | v4.8,65 3.7,66.1 2.56,66.1 K6.S2
  Bottom 0.508: v4.8,65 7.5,62.3 v7.5,45.1
SCLK_DAC  (via drill 0.5)
  Top(V+) 0.254: IC2.10 58.6,24 v58.2,24.4 | v58.1,13.7 58.6,13.2 IC3.10
  midBottom(V-) 0.305: v58.2,24.4 58.6,24 58.6,14.2 v58.1,13.7 58.1,7.5 59.5,6.1
  midBottom(V-) 0.406: 59.5,6.1 83,6.1 91.6,6.1 92.1,6.6 92.1,16.9 93.2,18 99.9,18 100.4,18.5 100.4,34.5 103.4,37.5 106.5,37.5 107.39,36.61 U1.CN12_25
SYM1  (via drill 0.5)
  Top(V+) 0.305: R39.2 R40.2 46.8,36.4
  Top(V+) 0.508: v46.8,37.8 46.8,36.4 | v57.95,67.95 58.1,67.8 VCA1(LEFT).4 | R40.2 R38.1
  Bottom 0.508: v46.8,37.8 46.45,38.15 46.45,69.8 56.2,69.8 58,68 v57.95,67.95
SYM2  (via drill 0.5)
  Top(V+) 0.305: R42.2 R43.2 48.1,32.2 R41.1
  Top(V+) 0.508: 48.1,32.2 48.1,33.5 v49.1,34.5 | v52.9,59.7 57.8,59.7 58.1,59.41 VCA2(RIGHT).4
  Bottom 0.508: v49.1,34.5 49.1,58.4 50.4,59.7 v52.9,59.7
SYM3  (via drill 0.5)
  Top(V+) 0.305: R44.1 R63.2 R45.2
  Top(V+) 0.508: R44.1 48.15,28.65 v49.2,29.7 | v36.9,46.7 36.9,47.2 35.99,48.1 STAGE(LEFT).4
  Bottom 0.508: v49.2,29.7 46.7,29.7 45.61,30.79 45.61,42.69 41.65,46.65 36.95,46.65 v36.9,46.7
SYM4  (via drill 0.5)
  Top(V+) 0.305: R65.2 R66.2 R64.1
  Top(V+) 0.508: R64.1 48.15,24.95 v49.1,25.9 | v36.8,38.7 36.8,39.2 35.99,40.01 STAGE(RIGHT).4
  Bottom 0.508: v49.1,25.9 44.7,30.3 44.7,37.2 43.2,38.7 v36.8,38.7
V+
  Top(V+) 0.406: OUT_RIGHT.6 17.6,79.17 C13.1 | 42.1,79.36 OUT_LEFT.6 | U$1.1 130.42,2.7 C101.1 128.65,3.95 127.8,4.8 125.8,4.8 125,4 125,2.5 124.8,2.3 23,2.3
  Top(V+) 0.508: C11.1 42.1,79.36 | C3.1 73.69,80.53 IN_RIGHT.7 | C1.1 96.22,80.85 IN_LEFT.7 | U4.7 96.31,67.75 98.5,67.75 C22.1 | U6.7 73.52,67.73 C26.1 | C5.1 IC4.8 | VCA1(LEFT).7 52.84,63.6 C62.1 | VCA2(RIGHT).7 51.02,55.37 C61.1 | IC8.8 60.05,48.91 C53.1 | C47.1 26.91,45.56 STAGE(LEFT).7 | C46.1 28.96,37.5 STAGE(RIGHT).7 | IC5.8 C35.1 | IC1.8 21.41,24.75 C7.1 | C28.1 14.38,37.45 U8.7 | C30.1 2.42,37.47 U7.7 | IC9.8 29.65,24.5 C58.1 | IC7.8 41.15,12.1 C49.1 | 23,2.3 19.91,5.39 CONN3.2
  pour Top(V+): 52.4,32.7 52.4,-1.3 -0.6,-1.3 -0.6,108.2 100,108.2 100,49 91.1,49 91.1,7.5 61.5,7.5 61.5,32.7
V-  (via drill 0.5)
  Top(V+) 0.254: R2.1 98.6,56 v98.7,56.1
  Top(V+) 0.305: R40.1 v43.7,36.4 | R43.1 v43.7,32.2 | R63.1 v43.7,28 | R66.1 v43.7,23.8
  Top(V+) 0.406: -15VOK.1 6.9,9.7 14.7,9.7 14.7,11.4 TP23.P$1
  Top(V+) 0.508: C14.1 v15.3,78.55 15.64,78.55 OUT_RIGHT.5 | OUT_LEFT.5 40.15,78.75 v39.7,78.75 C12.1 | IN_RIGHT.4 66.16,77.95 C4.1 65.8,77.95 v65.8,76.1 | C2.1 88.64,78.3 IN_LEFT.4 v91,76.6 | IC4.4 C6.1 85.65,67.05 v85.6,67 | v87,64.8 87.05,64.75 C21.1 90.66,64.75 U4.4 | U6.4 64.34,65.19 C25.1 v63.9,63.5 | R51.1 v47.6,57.9 | R50.1 v47.6,66.2 | IC8.4 51.35,45.09 | 51.35,45.09 C54.1 | 51.35,45.09 51.35,43.95 v51.4,43.9 | R31.1 v23.4,48.1 | R32.1 v23.5,40 | C36.1 28,28 | 28,28 IC5.4 | C8.1 17.05,31.5 IC1.4 17.59,33.49 v18.4,34.3 | C29.1 20.15,40.55 U8.4 v21.59,40.01 v21.6,40 | U7.4 10.55,40.76 C27.1 v11.7,42 | 28,28 28.9,27.1 v28.9,26.9 | C57.1 IC9.4 24.15,16.15 v24.1,16.1 | IC7.4 C50.1 35.55,5.3 v34.3,5.3
  pour midBottom(V-): 100,108.4 100,48.9 91,48.9 91,7.5 61.5,7.5 61.5,32.7 52.5,32.7 52.5,-2.1 -1.4,-2.1 -1.4,108.4

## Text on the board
tNames: AGND | quantum | AnalougeEngine / V4_0 | -15V | +15V | -15V | AGND | +15V | DGND | bottom | CHASIS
